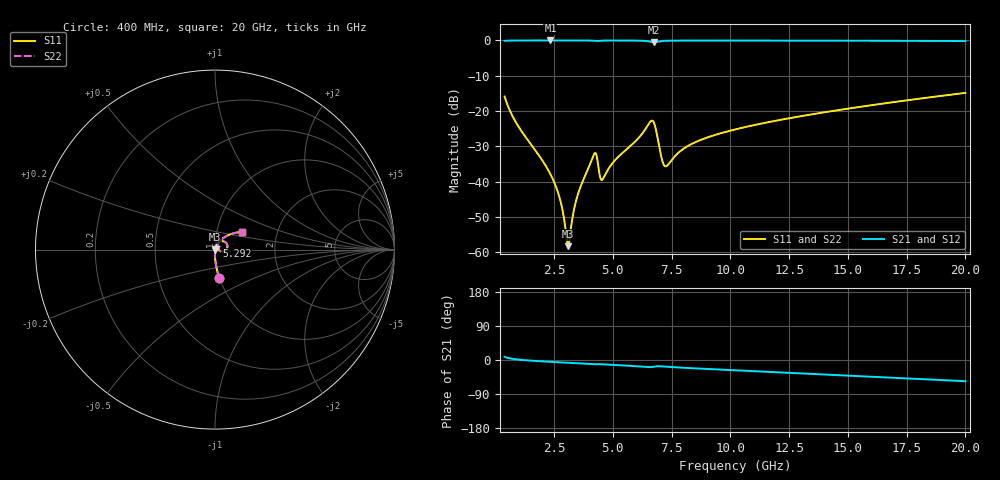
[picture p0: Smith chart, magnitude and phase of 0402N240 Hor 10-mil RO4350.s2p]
# GHz S MA R 50
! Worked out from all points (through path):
!   1960 points, 400 MHz to 20 GHz, reference 50 ohm
!   highest |S21| = -0.01 dB at 2.351 GHz (marker M1); lowest = -0.6 dB at 6.743 GHz (marker M2)
!   group delay of S21, straight-line fit = 8.08 ps
!   lowest |S11| = -58.3 dB at 3.101 GHz (marker M3), VSWR 1.00, Z = 50.1 - j0.0215 ohm
!   |S11| at or under -10 dB: start of sweep to end of sweep
!   |S22| runs from -58.3 to -14.9 dB; largest |S21 - S12| = 0
!   S11 on the Smith chart (normalised r, x): 400 MHz: 1.00, -0.32; 5.292 GHz: 1.02, +0.04; 20 GHz: 1.33, +0.27
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0.4  0.1605 -81.5  0.9865 8.3  0.9865 8.3  0.1605 -81.5
0.9302705  0.06496 -87.8  0.9971 1.5  0.9971 1.5  0.06496 -87.8
2.350995  0.01271 -90.2  0.9988 -4.9  0.9988 -4.9  0.01271 -90.2
2.7512  0.005717 -85.0  0.9988 -6.2  0.9988 -6.2  0.005717 -85.0
3.101378  0.001219 -10.2  0.9986 -7.4  0.9986 -7.4  0.001219 -10.2
3.401531  0.004789 64.9  0.9985 -8.3  0.9985 -8.3  0.004789 64.9
3.671669  0.009218 70.0  0.9981 -9.2  0.9981 -9.2  0.009218 70.0
4.211945  0.02477 47.5  0.9867 -11.2  0.9867 -11.2  0.02477 47.5
4.301991  0.02404 25.7  0.9804 -11.0  0.9804 -11.0  0.02404 25.7
4.462072  0.0116 22.9  0.9902 -11.0  0.9902 -11.0  0.0116 22.9
4.552118  0.01064 43.4  0.9936 -11.3  0.9936 -11.3  0.01064 43.4
5.292496  0.02339 69.8  0.9969 -13.9  0.9969 -13.9  0.02339 69.8
6.59316  0.07037 36.7  0.9583 -18.9  0.9583 -18.9  0.07037 36.7
6.743236  0.06919 8.8  0.9373 -17.7  0.9373 -17.7  0.06919 8.8
6.943338  0.03589 -15.9  0.9638 -16.4  0.9638 -16.4  0.03589 -15.9
7.12343  0.01896 0.0  0.9816 -17.2  0.9816 -17.2  0.01896 0.0
7.273507  0.01653 26.7  0.9878 -17.9  0.9878 -17.9  0.01653 26.7
8.304033  0.03348 62.3  0.9955 -21.5  0.9955 -21.5  0.03348 62.3
10.205  0.05484 60.2  0.9955 -27.1  0.9955 -27.1  0.05484 60.2
13.46667  0.08976 51.9  0.9929 -36.5  0.9929 -36.5  0.08976 51.9
16.73834  0.1309 42.7  0.988 -46.1  0.988 -46.1  0.1309 42.7
20  0.1807 33.1  0.9798 -56.0  0.9798 -56.0  0.1807 33.1
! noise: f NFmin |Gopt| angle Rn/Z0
0.4  0.001229  0.7809  1.238  0.00115
2.571  0.004358  0.6355  6.163  0.002245
4.752  0.01057  0.7106  11.23  0.00713
6.933  0.04193  0.8835  16.39  0.07646
9.104  0.01339  0.597  21.1  0.005919
11.29  0.01397  0.5422  25.71  0.005175
13.47  0.01541  0.5181  30.21  0.005248
15.64  0.01702  0.5045  34.55  0.005482
17.82  0.01871  0.4967  38.76  0.00578
20  0.02045  0.4931  42.82  0.006118
